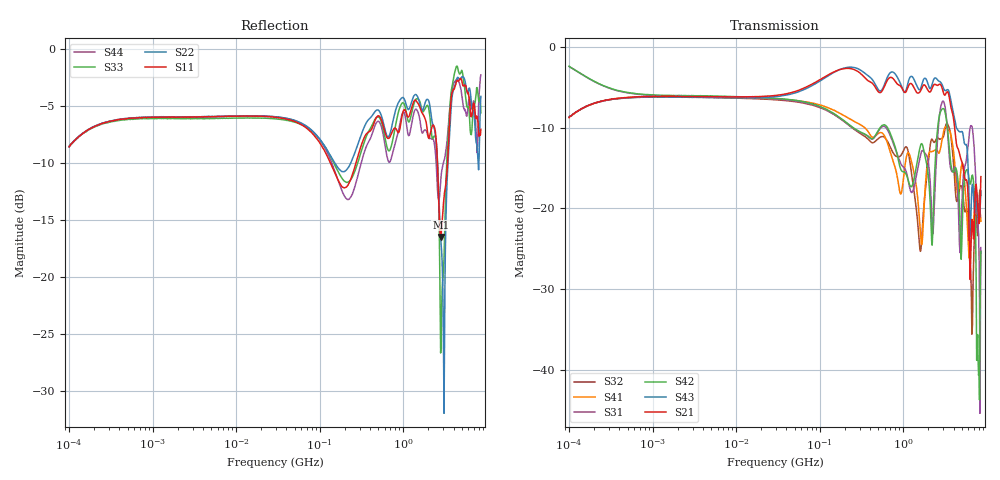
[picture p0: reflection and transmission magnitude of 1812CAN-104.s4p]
# Hz S dB R 50
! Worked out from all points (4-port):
!   801 points, 100 kHz to 8.5 GHz, reference 50 ohm
!   strongest paths, dB at 100 kHz, 1.721 MHz, 29.51 MHz, 502.3 MHz, 8.5 GHz:
!     S21: -8.8, -6.1, -6.0, -5.6, -16.1
!     S43: -8.7, -6.2, -6.2, -5.3, -17.9
!     S42: -2.4, -6.0, -6.4, -10.4, -25.4
!     S31: -2.4, -6.1, -6.5, -10.5, -24.9
!     S41: -8.8, -6.2, -6.4, -10.7, -21.6
!     S32: -8.7, -6.2, -6.6, -11.4, -18.4
!   lowest |S11| = -16.5 dB at 2.804 GHz (marker M1), VSWR 1.35, Z = 42.2 + j11.5 ohm
!   |S11| at or under -10 dB: 133.9 MHz to 272.7 MHz (138.8 MHz wide, 68.3 % of centre); 2.564 GHz to 3.394 GHz (829.8 MHz wide, 27.9 % of centre)
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100000  -8.62 40.5  -8.78 41.7  -2.45 -18.5  -8.78 -139.1
        -8.76 41.6  -8.61 40.1  -8.76 -138.5  -2.46 -18.6
        -2.45 -18.6  -8.72 -138.8  -8.58 40.9  -8.74 41.1
        -8.77 -138.7  -2.40 -18.7  -8.71 40.7  -8.60 40.8
1.48093e9  -4.74 53.5  -5.73 -12.7  -15.26 141.6  -18.62 -8.3
           -5.73 -12.6  -4.20 47.9  -21.56 12.4  -14.05 132.4
           -15.25 141.7  -21.51 12.6  -4.40 52.6  -4.99 -14.2
           -18.51 -8.5  -14.01 132.8  -4.99 -14.1  -5.47 57.5
2.804235e9  -16.53 117.0  -4.72 -28.5  -7.51 66.4  -12.46 38.0
            -4.69 -28.5  -16.52 76.3  -11.43 53.8  -8.04 52.5
            -7.50 66.3  -11.41 53.5  -26.71 104.9  -4.41 -27.6
            -12.50 37.9  -8.01 52.6  -4.39 -27.5  -11.63 142.2
5.086878e9  -3.02 -96.3  -14.37 -46.1  -18.22 52.4  -14.43 -51.1
            -14.39 -46.3  -2.45 -91.8  -17.61 -32.4  -22.04 31.0
            -18.29 52.2  -17.61 -32.8  -2.02 -101.4  -10.54 -42.1
            -14.41 -51.1  -22.07 31.6  -10.51 -41.9  -4.38 -108.7
6.842542e9  -5.00 12.3  -22.79 6.9  -10.75 -34.6  -22.31 139.3
            -22.74 6.8  -5.40 -3.0  -29.48 90.5  -16.24 -48.8
            -10.74 -34.9  -29.49 90.8  -5.38 26.7  -17.44 -23.0
            -22.32 139.6  -16.19 -48.5  -17.48 -22.7  -4.84 2.6
7.878453e9  -6.52 77.1  -20.47 19.0  -22.32 -74.4  -21.06 33.6
            -20.44 18.8  -9.93 75.7  -22.43 37.3  -38.77 -52.5
            -22.36 -74.8  -22.44 37.2  -4.08 80.2  -21.02 8.2
            -21.08 34.1  -38.94 -51.1  -21.02 8.7  -6.49 103.6
8.5e9  -7.08 136.0  -16.11 60.8  -24.94 62.6  -21.66 18.4
       -16.08 60.8  -4.20 134.4  -18.38 7.9  -25.28 61.8
       -24.87 62.7  -18.38 7.4  -5.63 120.4  -17.86 37.3
       -21.61 18.2  -25.36 61.8  -17.90 37.6  -2.30 126.6
